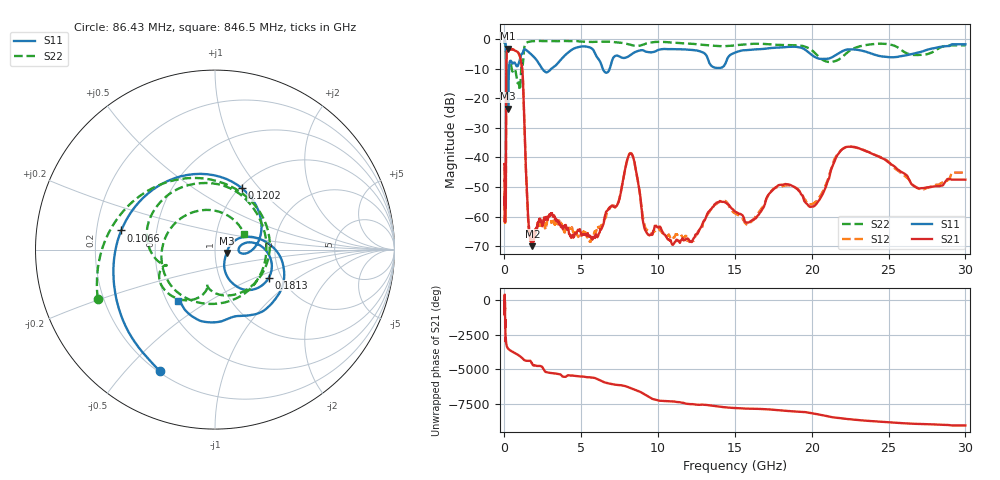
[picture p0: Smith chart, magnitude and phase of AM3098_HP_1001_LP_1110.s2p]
! Date/Time: Thu, Feb 28, 2019 8:41 AM
! Network Analyzer: Agilent Technologies E8364B Rev: A.07.50.67
! Sweep from 0.010 to 30.000 GHz, 1601 Points, Sweep Type: LOG
! Power Supply: 5.022 V, 0.002 A
# Hz S DB R 50
!freq MagS11 AngS11 MagS21 AngS21 MagS12 AngS12 MagS22 AngS22
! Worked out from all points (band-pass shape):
!   1601 points, 10 MHz to 30 GHz, reference 50 ohm
!   highest |S21| = -3.12 dB at 247.2 MHz (marker M1); lowest = -70.1 dB at 1.82 GHz (marker M2)
!   |S21| within 3 dB of the highest: 130.1 MHz to 1.027 GHz (896.6 MHz wide, 155 % of centre)
!   lowest |S11| = -23.5 dB at 239.9 MHz (marker M3), VSWR 1.14, Z = 56.8 - j2.22 ohm
!   |S11| at or under -10 dB: 192.4 MHz to 299.7 MHz (107.2 MHz wide, 43.6 % of centre); 2.474 GHz to 3.031 GHz (557.8 MHz wide, 20.3 % of centre); 6.403 GHz to 6.844 GHz (441.1 MHz wide, 6.66 % of centre)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
!   |S22| runs from -17.2 to -0.5 dB; largest |S21 - S12| = 0.014
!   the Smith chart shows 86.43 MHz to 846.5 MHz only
!   S11 on the Smith chart (normalised r, x): 86.43 MHz: 0.21, -0.63; 106.6 MHz: 0.31, +0.09; 120.2 MHz: 1.03, +0.81; 181.3 MHz: 1.72, -0.61; 846.5 MHz: 0.57, -0.38
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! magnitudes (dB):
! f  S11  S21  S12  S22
! 10 MHz  -0.3  -42.2  -42.9  -0.6
! 38.04 MHz  -0.5  -60.4  -62.4  -1.0
! 48.13 MHz  -0.7  -50.0  -50.1  -1.3
! 86.43 MHz  -2.6  -56.5  -56.8  -3.0
! 106.6 MHz  -5.5  -27.9  -27.7  -7.0
! 120.2 MHz  -8.6  -10.9  -10.9  -10.5
! 144.7 MHz  -17.3  -4.4  -4.4  -13.4
! 181.3 MHz  -9.4  -3.7  -3.7  -8.9
! 239.9 MHz  -23.5  -3.1  -3.1  -10.9
! 247.2 MHz  -22.0  -3.1  -3.1  -10.8
! 550.5 MHz  -8.1  -3.5  -3.4  -10.8
! 846.5 MHz  -9.1  -4.2  -4.2  -14.7
! 1.172 GHz  -4.8  -10.9  -10.8  -8.7
! 1.551 GHz  -4.2  -61.0  -62.2  -0.8
! 1.82 GHz  -5.4  -70.1  -67.9  -0.6
! 2.084 GHz  -6.9  -63.9  -64.2  -0.5
! 5.87 GHz  -4.4  -66.8  -65.0  -0.8
! 7.926 GHz  -6.1  -42.2  -42.2  -1.4
! 11.08 GHz  -3.3  -68.7  -66.9  -1.1
! 20.1 GHz  -5.6  -56.6  -55.6  -4.1
! 22.56 GHz  -3.3  -36.3  -36.4  -3.5
! 30 GHz  -1.6  -47.5  -45.1  -2.0
